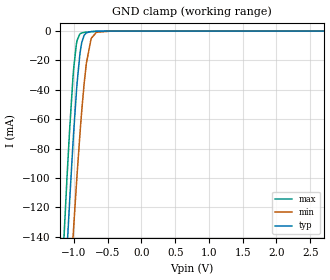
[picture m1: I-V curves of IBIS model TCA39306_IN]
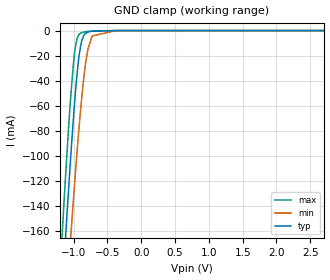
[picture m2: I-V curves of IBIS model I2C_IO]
|Texas Instruments Incorporated
| Low voltage FM+ I2C bus and SMBus voltage translator
| TCA39306
| Voltage Range : 0.9V-5.5V
| Package-type: DCU / DCT / DTM
| #pins/pkg drawing : 8-pin DCU /  8-pin DCT / 8-pin DTM
[IBIS Ver] 4.1
[File name] tca39306_1p5.ibs
[File Rev] 1.0
[Date] 07/01/2021
[Source]
| Texas Instruments Incorporated.
| 12500 TI Blvd
| Dallas, TX -75243
[Notes] Revision History:
| Rev 1.0: 07/01/2021
| - Initial version of the model
| - Model generated from simulations in SPECTRE
| - C_comp although listed in numerical order of value are
| obtained from varying PVT conditions. For PVT conditions for
| each specific value refer the buffer description under
| respective [Model]. IBIS model user is responsible for using
| appropriate C_comp to simulate for Signal Integrity.
| - Warnings regarding combined Non-monotonicity of various models have been
| reviewed and considered minor and can be ignored.
[Disclaimer]
| This model is designed as an aid for customers of Texas Instruments.
| TI and its licensors and suppliers make no warranties, either expressed
| or implied, with respect to this model, including the warranties of
| merchantability or fitness for a particular purpose. The model is
| provided solely on an "as is" basis. The entire risk as to its quality
| and performance is with the customer.
| This model is subject to change without notice. Texas Instruments
| Incorporated is not responsible for updating this model.
[Copyright]
(C) Copyright 2019 Texas Instruments Incorporated. All rights reserved.
| Component1 TCA39306DCU 8-PIN TSSOP
[Component] TCA39306_DCU
[Manufacturer] Texas Instruments Incorporated
[Package] |DCU 8-pin TSSOP
| variable typ   min   max
R_pkg 1.400e-02   1.300e-02   1.500e-02
L_pkg 1.289e-09   1.025e-09   2.014e-09
C_pkg 1.360e-13   6.600e-14   2.940e-13
[Pin]   signal_name   model_name   R_pin   L_pin   C_pin
1   GND   GND   1.400e-02   1.387e-09   1.760e-13
2   VREF1   I2C_IO   1.300e-02   1.026e-09   6.600e-14
3   SCL1   I2C_IO   1.300e-02   1.032e-09   6.700e-14
4   SDA1   I2C_IO   1.500e-02   2.014e-09   2.940e-13
5   SDA2   I2C_IO   1.400e-02   1.412e-09   1.780e-13
6   SCL2   I2C_IO   1.300e-02   1.030e-09   6.600e-14
7   VREF2   I2C_IO   1.300e-02   1.025e-09   6.600e-14
8   EN   TCA39306_IN   1.400e-02   1.386e-09   1.760e-13
[Series Pin Mapping]   pin_2   model_name   function_table_group
2   7   I2C_IO_S   1
3   6   I2C_IO_S   1
4   5   I2C_IO_S   1
[Series Switch Groups]
| Function Group States
On  1 /
Off 1 /
| Component2 TCA39306DCT 8-PIN TSSOP
[Component] TCA39306_DCT
[Manufacturer] Texas Instruments Incorporated
[Package] |DCU 8-pin TSSOP
| variable typ   min   max
R_pkg   2.900e-02   2.800e-02   3.100e-02
L_pkg   1.796e-09   1.666e-09   1.924e-09
C_pkg   1.090e-13   8.300e-14   1.360e-13
[Pin]   signal_name   model_name   R_pin   L_pin   C_pin
1   GND   GND   1.400e-02   1.387e-09   1.760e-13
2   VREF1   I2C_IO   1.300e-02   1.026e-09   6.600e-14
3   SCL1   I2C_IO   1.300e-02   1.032e-09   6.700e-14
4   SDA1   I2C_IO   1.500e-02   2.014e-09   2.940e-13
5   SDA2   I2C_IO   1.400e-02   1.412e-09   1.780e-13
6   SCL2   I2C_IO   1.300e-02   1.030e-09   6.600e-14
7   VREF2   I2C_IO   1.300e-02   1.025e-09   6.600e-14
8   EN   TCA39306_IN   1.400e-02   1.386e-09   1.760e-13
[Series Pin Mapping]   pin_2   model_name   function_table_group
2   7   I2C_IO_S   1
3   6   I2C_IO_S   1
4   5   I2C_IO_S   1
[Series Switch Groups]
| Function Group States
On 1 /
Off 1 /
| Component3 TCA39306DTM 8-PIN X2SON
[Component] TCA39306_DTM
[Manufacturer] Texas Instruments Incorporated
[Package] |DTM 8-pin X2SON
| variable typ   min   max
R_pkg   2.900e-02   2.800e-02   3.100e-02
L_pkg   1.796e-09   1.666e-09   1.924e-09
C_pkg   1.090e-13   8.300e-14   1.360e-13
[Pin]   signal_name   model_name   R_pin   L_pin   C_pin
1   GND   GND   3.000e-02   2.890e-10   7.058e-14
2   VREF1   I2C_IO   3.089e-02   2.672e-10   2.985e-13
3   SCL1   I2C_IO   3.203e-02   2.900e-10   .0654e-14
4   SDA1   I2C_IO   4.000e-02   4.124e-10   7.674e-13
5   SDA2   I2C_IO   3.190e-02   2.849e-10   1.780e-13
6   SCL2   I2C_IO   1.300e-02   2.664e-10   2.993e-13
7   VREF2   I2C_IO   3.206e-02   2.872e-10   6.541e-14
8   EN   TCA39306_IN   3.100e-02   2.839e-10   7.674e-13
[Series Pin Mapping]   pin_2   model_name   function_table_group
2   7   I2C_IO_S   1
3   6   I2C_IO_S   1
4   5   I2C_IO_S   1
[Series Switch Groups]
| Function Group States
On 1 /
Off 1 /
| I2C_IO_S
[Model]   I2C_IO_S
Model_type  Series_switch
| variable   typ   min   max
C_comp   2.6pF   2.2pF   3.5pF
[Temperature Range]   40   125   -40
[Voltage range]   1.5   1.35   1.65
[On]
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[Off]
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| Models and submodels in the file (3): TCA39306_IN (Input), I2C_IO_S (Series_switch), I2C_IO (Input)
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| TCA39306_IN
[Model]   TCA39306_IN
Model_type   Input
Vinl=0.9
Vinh=1.26
|   typ   min   max
C_comp   11pF   9.4pF   13pF
[Voltage Range]   1.5   1.35   1.65
[Temperature Range]   27   125   -40
[Power Clamp Reference]   1.8   1.62   1.98
[GND Clamp Reference]   0   0   0
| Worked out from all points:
|   GND clamp passes 1 mA (typ) near -0.80 V on its own axis
[GND Clamp]
|   Voltage   I(typ)   I(min)   I(max)
-1.8V     -816.2mA   -796.8mA   -796.5mA
-1.19V    -226.2mA   -277.8mA   -179.1mA
-1.103V   -149.2mA   -208.7mA   -100.1mA
-1.066V   -117.1mA   -179.4mA   -68.44mA
-1.006V   -70.4mA    -134.8mA   -26.8mA
-957.6mV  -37.91mA   -100.4mA   -7.316mA
-914.4mV  -16.76mA   -72.02mA   -2.128mA
-892.8mV  -9.89mA    -58.96mA   -1.415mA
-817.2mV  -1.2mA     -22.27mA   -706.6uA
-747mV    -309.3uA   -5.442mA   -430.6uA
-666mV    -106.5uA   -780.7uA   -203.8uA
3.6V      0A         0A         0A
| I2C_IO
[Model]   I2C_IO
Model_type   Input
Vinl = 0.45
Vinh = 1.05
|   typ   min   max
C_comp   2.6pF   2.2pF   3.5pF
[Voltage Range]   1.5   1.35   1.65
[Temperature Range]   27   125   -40
[Power Clamp Reference]   1.5   1.35   1.65
[GND Clamp Reference]   0   0   0
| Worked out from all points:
|   GND clamp passes 1 mA (typ) near -0.77 V on its own axis
[GND Clamp]
|   Voltage   I(typ)   I(min)   I(max)
-1.5V     -524.4mA   -541.3mA   -490.6mA
-1.257V   -290.7mA   -335.7mA   -245.9mA
-1.145V   -187.2mA   -243.7mA   -138.5mA
-1.113V   -159.3mA   -218.6mA   -110mA
-1.05V    -105.9mA   -169.6mA   -57.51mA
-1V       -67.66mA   -132.6mA   -24.72mA
-946.5mV  -32.87mA   -94.58mA   -6.007mA
-897mV    -12.1mA    -63.01mA   -2.054mA
-825mV    -2.205mA   -26.59mA   -911.8uA
-726mV    -486uA     -4.306mA   -368.1uA
-375mV    -361.9nA   -9.242uA   -501.1nA
3V        0A         0A         0A
